{attribute 'no_assign'}
FUNCTION_BLOCK FB_LD_IEDMUnn EXTENDS FB_AcsiCommonLogicalDeviceClass
VAR_INPUT
	LLN0: FB_LN_IED_MUnn_LLN0 := (sClass:='LLN0', bLinkResult:=THIS^.AddLogicalNodeToContainer(ipLogicalNode:=LLN0));
	LPHD1: FB_LN_IED_MUnn_LPHD1 := (sClass:='LPHD', bLinkResult:=THIS^.AddLogicalNodeToContainer(ipLogicalNode:=LPHD1));
	InnATCTR1: FB_LN_IED_MUnn_InnATCTR1 := (sClass:='TCTR', bLinkResult:=THIS^.AddLogicalNodeToContainer(ipLogicalNode:=InnATCTR1)); (*Current transformer*)
	InnBTCTR2: FB_LN_IED_MUnn_InnATCTR1 := (sClass:='TCTR', bLinkResult:=THIS^.AddLogicalNodeToContainer(ipLogicalNode:=InnBTCTR2)); (*Current transformer*)
	InnCTCTR3: FB_LN_IED_MUnn_InnATCTR1 := (sClass:='TCTR', bLinkResult:=THIS^.AddLogicalNodeToContainer(ipLogicalNode:=InnCTCTR3)); (*Current transformer*)
	InnNTCTR4: FB_LN_IED_MUnn_InnATCTR1 := (sClass:='TCTR', bLinkResult:=THIS^.AddLogicalNodeToContainer(ipLogicalNode:=InnNTCTR4)); (*Current transformer*)
	UnnATVTR1: FB_LN_IED_MUnn_UnnATVTR1 := (sClass:='TVTR', bLinkResult:=THIS^.AddLogicalNodeToContainer(ipLogicalNode:=UnnATVTR1)); (*Voltage transformer*)
	UnnBTVTR2: FB_LN_IED_MUnn_UnnATVTR1 := (sClass:='TVTR', bLinkResult:=THIS^.AddLogicalNodeToContainer(ipLogicalNode:=UnnBTVTR2)); (*Voltage transformer*)
	UnnCTVTR3: FB_LN_IED_MUnn_UnnATVTR1 := (sClass:='TVTR', bLinkResult:=THIS^.AddLogicalNodeToContainer(ipLogicalNode:=UnnCTVTR3)); (*Voltage transformer*)
	UnnNTVTR4: FB_LN_IED_MUnn_UnnATVTR1 := (sClass:='TVTR', bLinkResult:=THIS^.AddLogicalNodeToContainer(ipLogicalNode:=UnnNTVTR4)); (*Voltage transformer*)
END_VAR
VAR
END_VAR

END_FUNCTION_BLOCK
